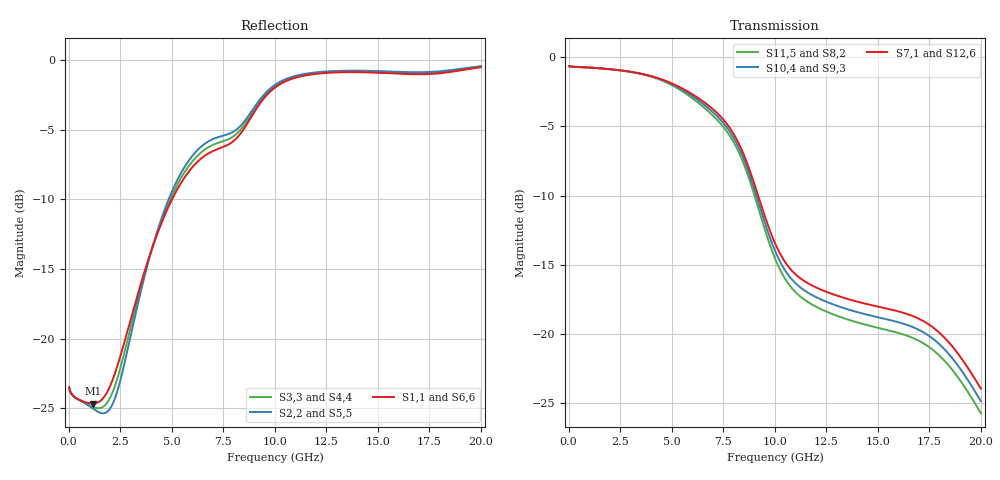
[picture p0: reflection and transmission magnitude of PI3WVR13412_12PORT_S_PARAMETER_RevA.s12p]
! NPort=12 DATA=800 NOISE=0 GROUPDELAY=0 COMPLEX_DATAFORMAT=POLAR
! NumOfBlock=1 NumOfParam=0
! .MODEL Smodel S TSTONEFILE=PI3WVR13412_12PORT_S_PARAMETER_RevA.s12p TYPE=S
!  -- The above .MODEL line can be used for the S element in the netlist.
! PORT DEFINITION
! PORT1 = INPUT1+
! PORT2 = INPUT1-
! PORT3 = INPUT2+
! PORT4 = INPUT2-
! PORT5 = INPUT3+
! PORT6 = INPUT3-
! PORT7 = OUTPUT1+
! PORT8 = OUTPUT1-
! PORT9 = OUTPUT2+
! PORT10 = OUTPUT2-
! PORT11 = OUTPUT3+
! PORT12 = OUTPUT3-
# Hz S MA R  50
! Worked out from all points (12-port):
!   800 points, 25 MHz to 20 GHz, reference 50 ohm
!   strongest paths, dB at 25 MHz, 5.025 GHz, 10.03 GHz, 15.03 GHz, 20 GHz:
!     S7,1: -0.6, -1.9, -13.5, -18.0, -24.0
!     S12,6: -0.6, -1.9, -13.5, -18.1, -24.0
!     S10,4: -0.6, -1.9, -14.0, -18.8, -24.9
!     S9,3: -0.6, -1.9, -14.0, -18.8, -24.9
!     S11,5: -0.6, -2.0, -14.6, -19.6, -25.8
!     S8,2: -0.6, -2.0, -14.6, -19.6, -25.8
!   lowest |S11| = -24.7 dB at 1.175 GHz (marker M1), VSWR 1.12, Z = 56.1 - j0.829 ohm
!   |S11| at or under -10 dB: start of sweep to 5.017 GHz
